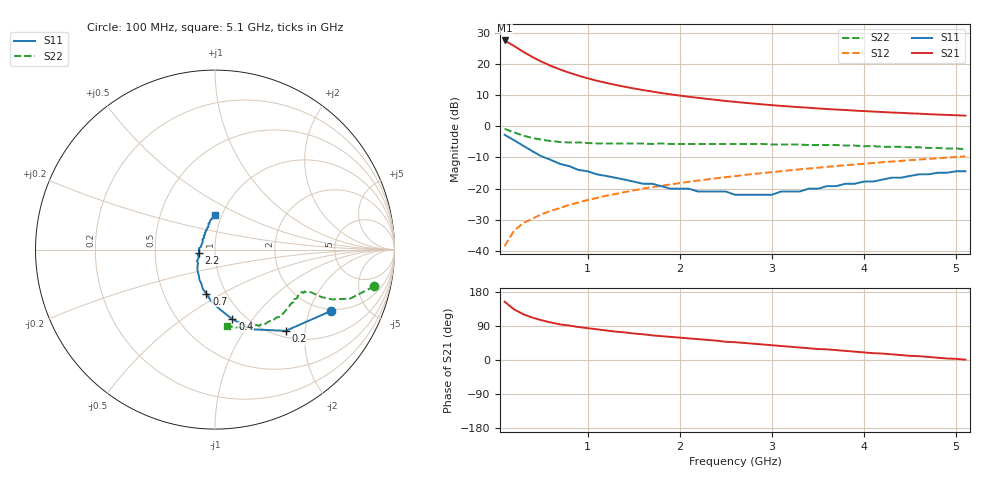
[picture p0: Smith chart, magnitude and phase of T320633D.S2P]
!AT-32063
!S PARAMETERS per side at Vce=2.7 V  Ic=10mA.  LAST UPDATED 08-19-96
# ghz s ma r 50
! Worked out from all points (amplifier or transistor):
!   51 points, 100 MHz to 5.1 GHz, reference 50 ohm
!   highest |S21| = 27.5 dB at 100 MHz (marker M1)
!   |S21| within 3 dB of that: start of sweep to 268.8 MHz
!   unconditionally stable (mu >= 1): 835.9 MHz to 4.317 GHz
!   at 900 MHz: K = 1.02, MAG = 19.6 dB, |S12| = -24.4 dB
!   at 2.6 GHz: K = 1.08, MAG = 10.1 dB, |S12| = -16.0 dB
!   at 5.1 GHz: K = 0.97, MSG = 6.5 dB, |S12| = -9.6 dB
!   S11 on the Smith chart (normalised r, x): 100 MHz: 1.92, -2.81; 200 MHz: 1.12, -1.58; 400 MHz: 0.87, -0.80; 700 MHz: 0.81, -0.42; 2.2 GHz: 0.84, -0.03; 5.1 GHz: 0.93, +0.37
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0.1  0.73 -28.0  23.69 154.0  0.012 76.0  0.91 -13.0
0.2  0.6 -49.0  19.43 134.0  0.021 69.0  0.8 -20.0
0.3  0.49 -65.0  15.69 121.0  0.028 66.0  0.71 -23.0
0.4  0.4 -76.0  12.9 112.0  0.033 65.0  0.65 -24.0
0.5  0.33 -86.0  10.84 105.0  0.039 64.0  0.61 -24.0
0.6  0.29 -94.0  9.3 99.0  0.044 65.0  0.58 -24.0
0.7  0.25 -101.0  8.14 94.0  0.049 65.0  0.56 -25.0
0.8  0.23 -107.0  7.22 91.0  0.055 65.0  0.55 -25.0
0.9  0.2 -113.0  6.48 87.0  0.06 65.0  0.55 -26.0
1  0.19 -117.0  5.87 84.0  0.066 66.0  0.54 -26.0
1.1  0.17 -122.0  5.37 81.0  0.071 65.0  0.53 -27.0
1.3  0.15 -131.0  4.61 75.0  0.082 65.0  0.53 -28.0
1.5  0.13 -138.0  4.04 70.0  0.094 64.0  0.53 -30.0
1.8  0.11 -150.0  3.41 63.0  0.111 62.0  0.53 -33.0
2.2  0.09 -169.0  2.85 55.0  0.135 59.0  0.52 -38.0
2.5  0.09 175.0  2.54 48.0  0.153 57.0  0.52 -42.0
2.6  0.08 170.0  2.46 47.0  0.159 56.0  0.52 -43.0
3  0.08 148.0  2.18 39.0  0.184 53.0  0.51 -48.0
3.1  0.09 141.0  2.12 37.0  0.191 52.0  0.51 -49.0
3.5  0.1 124.0  1.93 29.0  0.217 48.0  0.5 -54.0
4.3  0.15 104.0  1.66 15.0  0.272 39.0  0.47 -66.0
5.1  0.19 90.0  1.48 1.0  0.33 30.0  0.43 -81.0
